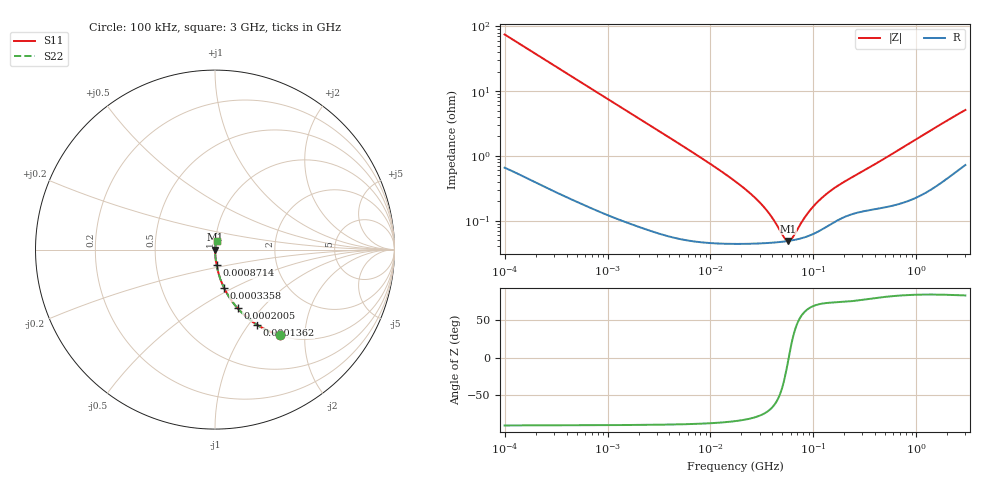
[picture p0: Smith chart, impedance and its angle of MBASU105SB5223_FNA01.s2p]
! MBASU105SB5223_FNA01  S-PARAMETER MODEL  ( Standard Model )
! Model Generated by TAIYO YUDEN Corporation (http://www.ty-top.com)
! Version 1.0
! TAIYO YUDEN Control No. 220601
! Copyright(c) 2014 TAIYO YUDEN CO.,LTD. All Rights Reserved.
! Product Description (link to TY-COMPAS)
! https://ds.yuden.co.jp/TYCOMPAS/or/detail?pn=MBASU105SB5223KFNA01&u=M
! Products Name : Multilayer Ceramic Capacitors
! Characteristics :
!  Capacitance : 0.022 [uF] , Rated Voltage : 50 [V] , TCC : X5R
!  Case Size : 1.0 x 0.5 / 0.039 x 0.02 [mm/inch] , Thickness : 0.5 / 0.02 [mm/inch]
!  (Conditions: Temperature = 25 [degC] , DC Bias Voltage = 0 [V])
! External Node Assignments :
!  1  o---| |---o  2
! GND o---------o GND
! Frequency Range : 100kHz  -  3GHz  [ 401 STEP ]
# MHZ S RI R 50
! Freq[MHz].  S11 Real  S11 Imag  S21 Real  S21 Imag  S12 Real  S12 Imag  S22 Real  S22 Imag
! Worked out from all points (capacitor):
!   401 points, 100 kHz to 3 GHz, reference 50 ohm
!   read as one part in series: C = 21.2 nF near 105.3 kHz
!   lowest |Z| = 48.6 mohm at 56.68 MHz (marker M1)
!   series resonance near 57.64 MHz, so ESL is about 360 pH
!   S11 on the Smith chart (normalised r, x): 100 kHz: 1.01, -1.50; 136.2 kHz: 1.01, -1.10; 200.5 kHz: 1.01, -0.75; 335.8 kHz: 1.01, -0.45; 871.4 kHz: 1.00, -0.17; 3 GHz: 1.01, +0.10
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0.1  0.36 -0.4756  0.64 0.4756  0.64 0.4756  0.36 -0.4756
0.136243  0.2345 -0.4189  0.7655 0.4189  0.7655 0.4189  0.2345 -0.4189
0.200542  0.1256 -0.3263  0.8744 0.3263  0.8744 0.3263  0.1256 -0.3263
0.335785  0.0502 -0.2126  0.9498 0.2126  0.9498 0.2126  0.0502 -0.2126
0.562235  0.0195 -0.1317  0.9805 0.1317  0.9805 0.1317  0.0195 -0.1317
0.871356  0.00882 -0.0862  0.9912 0.0862  0.9912 0.0862  0.00882 -0.0862
3.161081  0.00121 -0.0241  0.9988 0.0241  0.9988 0.0241  0.00121 -0.0241
9.331111  0.000517 -0.00802  0.9995 0.00802  0.9995 0.00802  0.000517 -0.00802
17.7727  0.000451 -0.00391  0.9995 0.00391  0.9995 0.00391  0.000451 -0.00391
24.84619  0.000445 -0.00252  0.9996 0.00252  0.9996 0.00252  0.000445 -0.00252
32.15051  0.000448 -0.00164  0.9996 0.00164  0.9996 0.00164  0.000448 -0.00164
39.51212  0.000456 -0.00103  0.9995 0.00103  0.9995 0.00103  0.000456 -0.00103
52.46276  0.000475 -0.000251  0.9995 0.000251  0.9995 0.000251  0.000475 -0.000251
56.67997  0.000483 -4.46e-05  0.9995 4.46e-05  0.9995 4.46e-05  0.000483 -4.46e-05
59.67813  0.000489 9.27e-05  0.9995 -9.27e-05  0.9995 -9.27e-05  0.000489 9.27e-05
62.83488  0.000496 0.00023  0.9995 -0.00023  0.9995 -0.00023  0.000496 0.00023
81.30716  0.000549 0.000934  0.9995 -0.000934  0.9995 -0.000934  0.000549 0.000934
97.38194  0.000612 0.00145  0.9994 -0.00145  0.9994 -0.00145  0.000612 0.00145
122.8043  0.000742 0.00217  0.9993 -0.00217  0.9993 -0.00217  0.000742 0.00217
163.0551  0.000971 0.00309  0.999 -0.00309  0.999 -0.00309  0.000971 0.00309
547.5153  0.00175 0.00991  0.9983 -0.00991  0.9983 -0.00991  0.00175 0.00991
3000  0.00966 0.0497  0.9903 -0.0497  0.9903 -0.0497  0.00966 0.0497
